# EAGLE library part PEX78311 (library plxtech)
PCI Express Endpoint Interface Auto generated by make-symbol-device-package-bsdl.ulp Rev. 16 from PEX8311_BSDL_netlist_r1.0.dat and manuell corrected Source: PEX_8311AA_Data_Book_v0.90_10Apr06.pdf
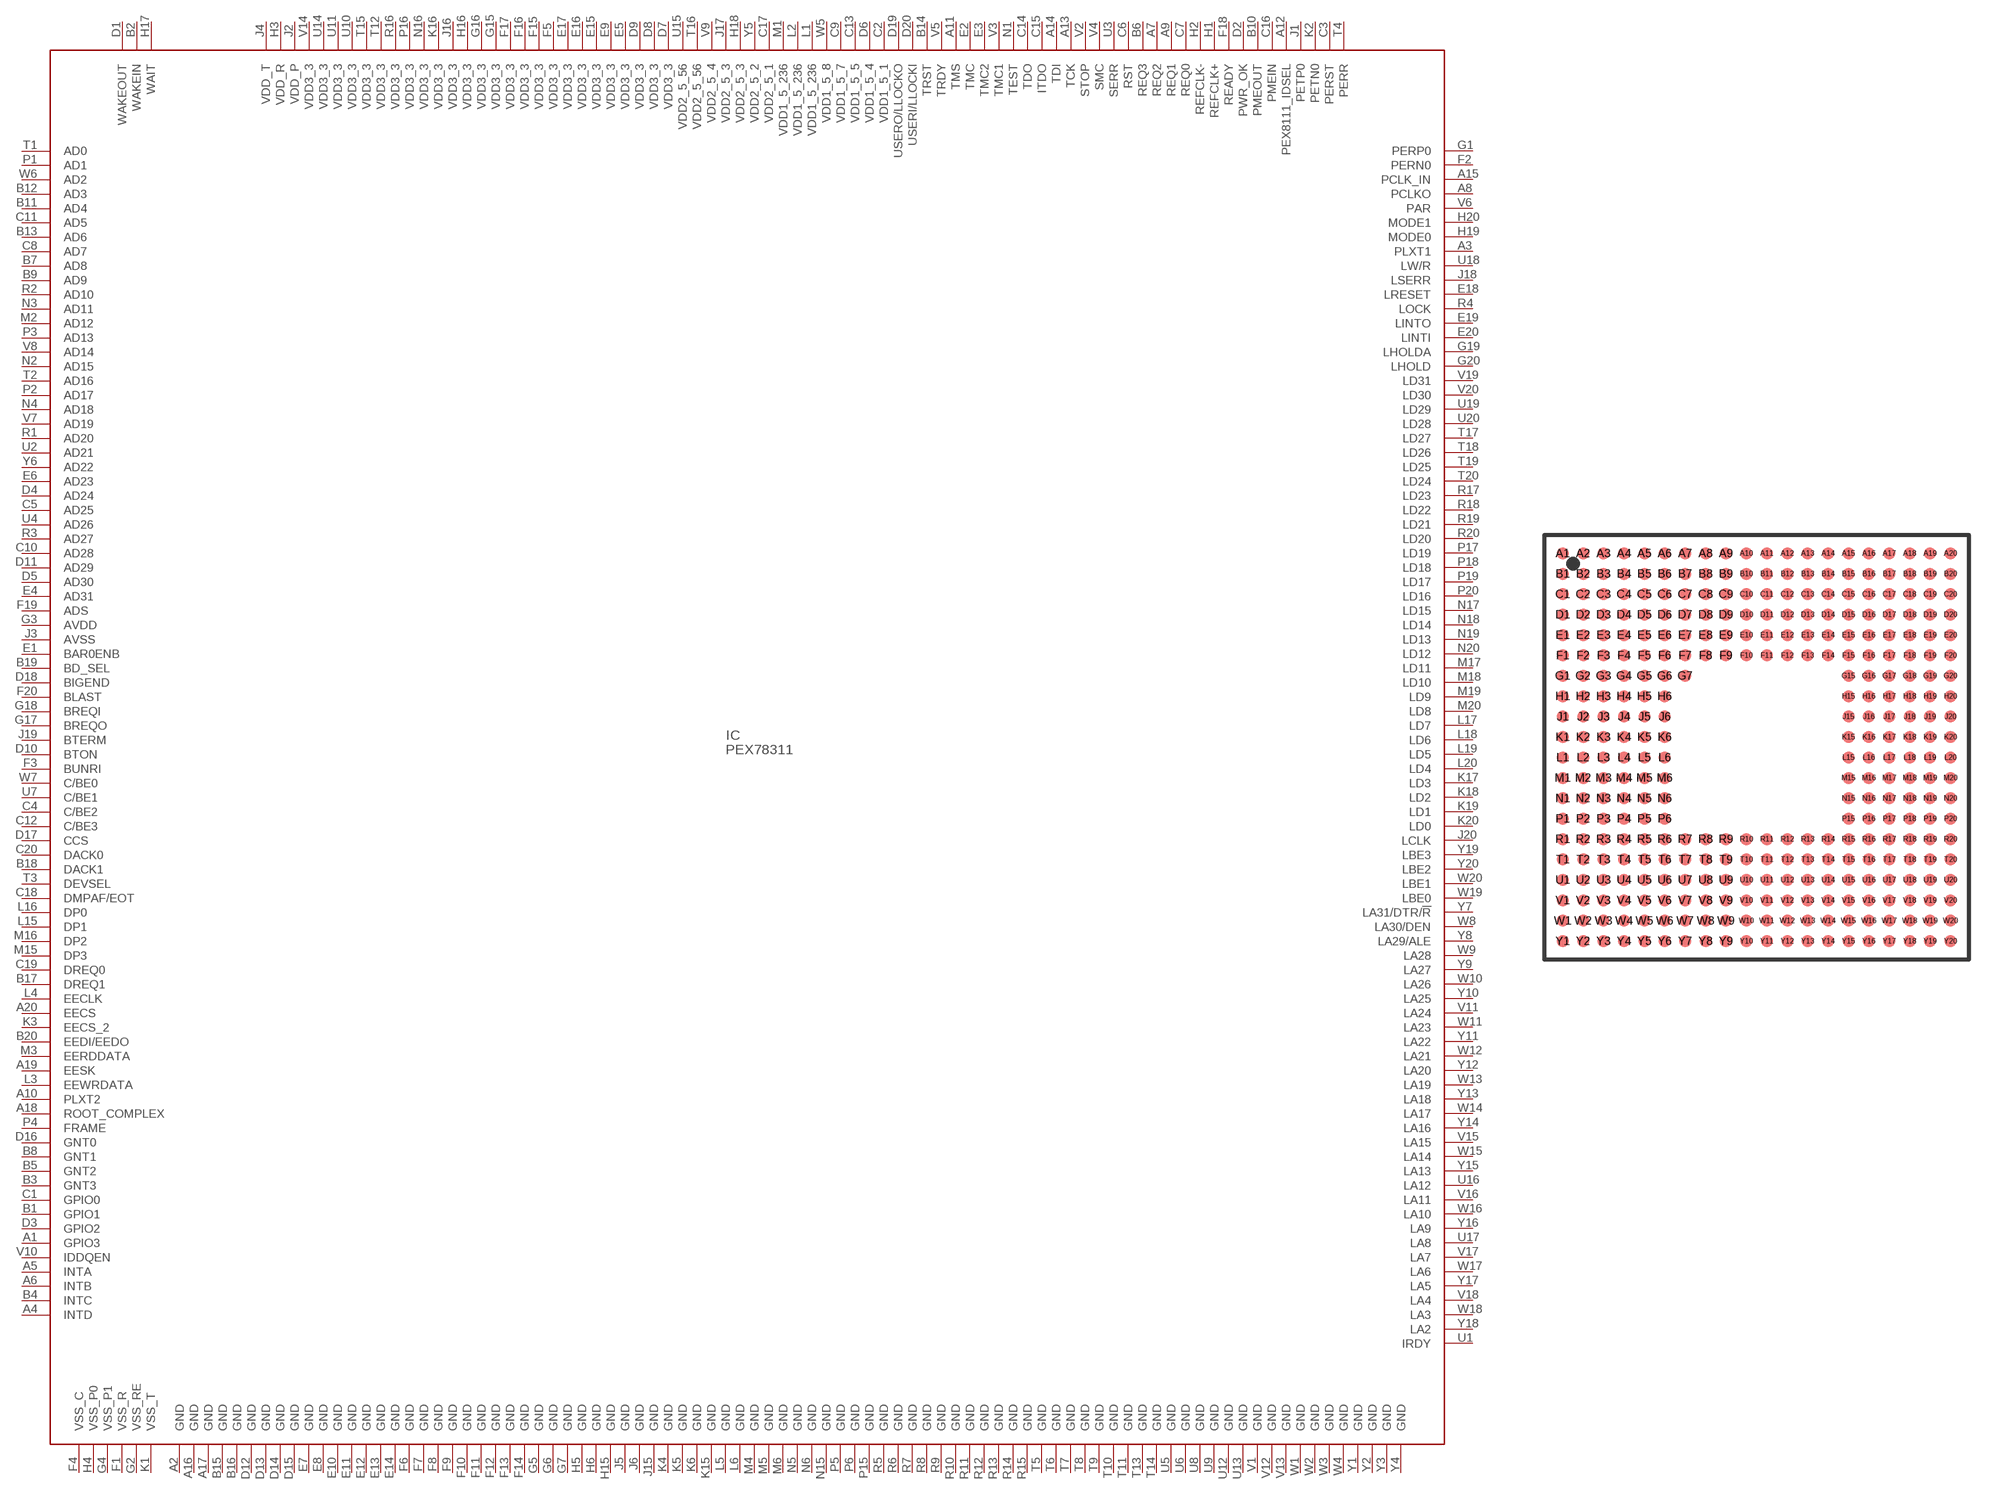
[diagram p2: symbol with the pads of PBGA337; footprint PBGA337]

Designator prefix IC

## PEX78311 (OC_FARNELL: unknown; OC_NEWARK: unknown)  [PBGA337]
A1  GPIO3
A2  GND  pwr
A3  PLXT1  in
A4  INTD
A5  INTA
A6  INTB
A7  REQ2
A8  PCLKO  out
A9  REQ1
A10  PLXT2  in
A11  TMS  in
A12  PEX8111_IDSEL
A13  TCK  in
A14  TDI  in
A15  PCLK_IN  in
A16  GND  pwr
A17  GND  pwr
A18  ROOT_COMPLEX  in
A19  EESK  out
A20  EECS  out
B1  GPIO1
B2  WAKEIN  in
B3  GNT3
B4  INTC
B5  GNT2
B6  REQ3
B7  AD8
B8  GNT1
B9  AD9
B10  PMEOUT  out
B11  AD4
B12  AD3
B13  AD6
B14  TRST  in
B15  GND  pwr
B16  GND  pwr
B17  DREQ1  in
B18  DACK1  out
B19  BD_SEL  in
B20  EEDI/EEDO
C1  GPIO0
C2  VDD1_5_1  pwr
C3  PERST
C4  C/BE2
C5  AD25
C6  RST
C7  REQ0
C8  AD7
C9  VDD1_5_7  pwr
C10  AD28
C11  AD5
C12  C/BE3
C13  VDD1_5_5  pwr
C14  TDO  out
C15  ITDO
C16  PMEIN  in
C17  VDD2_5_1  pwr
C18  DMPAF/EOT
C19  DREQ0  in
C20  DACK0  out
D1  WAKEOUT  out
D2  PWR_OK  out
D3  GPIO2
D4  AD24
D5  AD30
D6  VDD1_5_4  pwr
D7  VDD3_3  pwr
D8  VDD3_3  pwr
D9  VDD3_3  pwr
D10  BTON  in
D11  AD29
D12  GND  pwr
D13  GND  pwr
D14  GND  pwr
D15  GND  pwr
D16  GNT0
D17  CCS  in
D18  BIGEND  in
D19  USERO/LLOCKO  out
D20  USERI/LLOCKI  in
E1  BAR0ENB  in
E2  TMC  in
E3  TMC2  in
E4  AD31
E5  VDD3_3  pwr
E6  AD23
E7  GND  pwr
E8  GND  pwr
E9  VDD3_3  pwr
E10  GND  pwr
E11  GND  pwr
E12  GND  pwr
E13  GND  pwr
E14  GND  pwr
E15  VDD3_3  pwr
E16  VDD3_3  pwr
E17  VDD3_3  pwr
E18  LRESET
E19  LINTO  out
E20  LINTI  in
F1  VSS_R  pwr
F2  PERN0  in
F3  BUNRI  in
F4  VSS_C  pwr
F5  VDD3_3  pwr
F6  GND  pwr
F7  GND  pwr
F8  GND  pwr
F9  GND  pwr
F10  GND  pwr
F11  GND  pwr
F12  GND  pwr
F13  GND  pwr
F14  GND  pwr
F15  VDD3_3  pwr
F16  VDD3_3  pwr
F17  VDD3_3  pwr
F18  READY
F19  ADS
F20  BLAST
G1  PERP0  in
G2  VSS_RE  pwr
G3  AVDD  pwr
G4  VSS_P1  pwr
G5  GND  pwr
G6  GND  pwr
G7  GND  pwr
G15  VDD3_3  pwr
G16  VDD3_3  pwr
G17  BREQO  out
G18  BREQI  in
G19  LHOLDA  in
G20  LHOLD  out
H1  REFCLK+  in
H2  REFCLK-  in
H3  VDD_R  pwr
H4  VSS_P0  pwr
H5  GND  pwr
H6  GND  pwr
H15  GND  pwr
H16  VDD3_3  pwr
H17  WAIT
H18  VDD2_5_3  pwr
H19  MODE0  in
H20  MODE1  in
J1  PETP0  out
J2  VDD_P  pwr
J3  AVSS  pwr
J4  VDD_T  pwr
J5  GND  pwr
J6  GND  pwr
J15  GND  pwr
J16  VDD3_3  pwr
J17  VDD2_5_3  pwr
J18  LSERR  out
J19  BTERM
J20  LCLK  in
K1  VSS_T  pwr
K2  PETN0  out
K3  EECS_2
K4  GND  pwr
K5  GND  pwr
K6  GND  pwr
K15  GND  pwr
K16  VDD3_3  pwr
K17  LD3
K18  LD2
K19  LD1
K20  LD0
L1  VDD1_5_236  pwr
L2  VDD1_5_236  pwr
L3  EEWRDATA
L4  EECLK  out
L5  GND  pwr
L6  GND  pwr
L15  DP1
L16  DP0
L17  LD7
L18  LD6
L19  LD5
L20  LD4
M1  VDD1_5_236  pwr
M2  AD12
M3  EERDDATA  out
M4  GND  pwr
M5  GND  pwr
M6  GND  pwr
M15  DP3
M16  DP2
M17  LD11
M18  LD10
M19  LD9
M20  LD8
N1  TEST  in
N2  AD15
N3  AD11
N4  AD18
N5  GND  pwr
N6  GND  pwr
N15  GND  pwr
N16  VDD3_3  pwr
N17  LD15
N18  LD14
N19  LD13
N20  LD12
P1  AD1
P2  AD17
P3  AD13
P4  FRAME
P5  GND  pwr
P6  GND  pwr
P15  GND  pwr
P16  VDD3_3  pwr
P17  LD19
P18  LD18
P19  LD17
P20  LD16
R1  AD20
R2  AD10
R3  AD27
R4  LOCK
R5  GND  pwr
R6  GND  pwr
R7  GND  pwr
R8  GND  pwr
R9  GND  pwr
R10  GND  pwr
R11  GND  pwr
R12  GND  pwr
R13  GND  pwr
R14  GND  pwr
R15  GND  pwr
R16  VDD3_3  pwr
R17  LD23
R18  LD22
R19  LD21
R20  LD20
T1  AD0
T2  AD16
T3  DEVSEL
T4  PERR
T5  GND  pwr
T6  GND  pwr
T7  GND  pwr
T8  GND  pwr
T9  GND  pwr
T10  GND  pwr
T11  GND  pwr
T12  VDD3_3  pwr
T13  GND  pwr
T14  GND  pwr
T15  VDD3_3  pwr
T16  VDD2_5_56  pwr
T17  LD27
T18  LD26
T19  LD25
T20  LD24
U1  IRDY
U2  AD21
U3  SERR
U4  AD26
U5  GND  pwr
U6  GND  pwr
U7  C/BE1
U8  GND  pwr
U9  GND  pwr
U10  VDD3_3  pwr
U11  VDD3_3  pwr
U12  GND  pwr
U13  GND  pwr
U14  VDD3_3  pwr
U15  VDD2_5_56  pwr
U16  LA12
U17  LA8
U18  LW/R
U19  LD29
U20  LD28
V1  GND  pwr
V2  STOP
V3  TMC1  in
V4  SMC  in
V5  TRDY
V6  PAR
V7  AD19
V8  AD14
V9  VDD2_5_4  pwr
V10  IDDQEN  in
V11  LA24
V12  GND  pwr
V13  GND  pwr
V14  VDD3_3  pwr
V15  LA15
V16  LA11
V17  LA7
V18  LA4
V19  LD31
V20  LD30
W1  GND  pwr
W2  GND  pwr
W3  GND  pwr
W4  GND  pwr
W5  VDD1_5_8  pwr
W6  AD2
W7  C/BE0
W8  LA30/DEN
W9  LA28
W10  LA26
W11  LA23
W12  LA21
W13  LA19
W14  LA17
W15  LA14
W16  LA10
W17  LA6
W18  LA3
W19  LBE0
W20  LBE1
Y1  GND  pwr
Y2  GND  pwr
Y3  GND  pwr
Y4  GND  pwr
Y5  VDD2_5_2  pwr
Y6  AD22
Y7  LA31/DTR/!R
Y8  LA29/ALE
Y9  LA27
Y10  LA25
Y11  LA22
Y12  LA20
Y13  LA18
Y14  LA16
Y15  LA13
Y16  LA9
Y17  LA5
Y18  LA2
Y19  LBE3
Y20  LBE2

## Footprint PBGA337 (pad centres in mm)
PEX 8311 337-Ball PBGA Package Source: www.plxtech.com ... PEX_8311AA_Data_Book_v0.90_10Apr06.pdf
smd 0.6 x 0.6: A1 -9.5,9.5; A2 -8.5,9.5; A3 -7.5,9.5; A4 -6.5,9.5; A5 -5.5,9.5; A6 -4.5,9.5; A7 -3.5,9.5; A8 -2.5,9.5; A9 -1.5,9.5; A10 -0.5,9.5; A11 0.5,9.5; A12 1.5,9.5; A13 2.5,9.5; A14 3.5,9.5; A15 4.5,9.5; A16 5.5,9.5; A17 6.5,9.5; A18 7.5,9.5; A19 8.5,9.5; A20 9.5,9.5; B1 -9.5,8.5; B2 -8.5,8.5; B3 -7.5,8.5; B4 -6.5,8.5; B5 -5.5,8.5; B6 -4.5,8.5; B7 -3.5,8.5; B8 -2.5,8.5; B9 -1.5,8.5; B10 -0.5,8.5; B11 0.5,8.5; B12 1.5,8.5; B13 2.5,8.5; B14 3.5,8.5; B15 4.5,8.5; B16 5.5,8.5; B17 6.5,8.5; B18 7.5,8.5; B19 8.5,8.5; B20 9.5,8.5; C1 -9.5,7.5; C2 -8.5,7.5; C3 -7.5,7.5; C4 -6.5,7.5; C5 -5.5,7.5; C6 -4.5,7.5; C7 -3.5,7.5; C8 -2.5,7.5; C9 -1.5,7.5; C10 -0.5,7.5; C11 0.5,7.5; C12 1.5,7.5; C13 2.5,7.5; C14 3.5,7.5; C15 4.5,7.5; C16 5.5,7.5; C17 6.5,7.5; C18 7.5,7.5; C19 8.5,7.5; C20 9.5,7.5; D1 -9.5,6.5; D2 -8.5,6.5; D3 -7.5,6.5; D4 -6.5,6.5; D5 -5.5,6.5; D6 -4.5,6.5; D7 -3.5,6.5; D8 -2.5,6.5; D9 -1.5,6.5; D10 -0.5,6.5; D11 0.5,6.5; D12 1.5,6.5; D13 2.5,6.5; D14 3.5,6.5; D15 4.5,6.5; D16 5.5,6.5; D17 6.5,6.5; D18 7.5,6.5; D19 8.5,6.5; D20 9.5,6.5; E1 -9.5,5.5; E2 -8.5,5.5; E3 -7.5,5.5; E4 -6.5,5.5; E5 -5.5,5.5; E6 -4.5,5.5; E7 -3.5,5.5; E8 -2.5,5.5; E9 -1.5,5.5; E10 -0.5,5.5; E11 0.5,5.5; E12 1.5,5.5; E13 2.5,5.5; E14 3.5,5.5; E15 4.5,5.5; E16 5.5,5.5; E17 6.5,5.5; E18 7.5,5.5; E19 8.5,5.5; E20 9.5,5.5; F1 -9.5,4.5; F2 -8.5,4.5; F3 -7.5,4.5; F4 -6.5,4.5; F5 -5.5,4.5; F6 -4.5,4.5; F7 -3.5,4.5; F8 -2.5,4.5; F9 -1.5,4.5; F10 -0.5,4.5; F11 0.5,4.5; F12 1.5,4.5; F13 2.5,4.5; F14 3.5,4.5; F15 4.5,4.5; F16 5.5,4.5; F17 6.5,4.5; F18 7.5,4.5; F19 8.5,4.5; F20 9.5,4.5; G1 -9.5,3.5; G2 -8.5,3.5; G3 -7.5,3.5; G4 -6.5,3.5; G5 -5.5,3.5; G6 -4.5,3.5; G7 -3.5,3.5; G15 4.5,3.5; G16 5.5,3.5; G17 6.5,3.5; G18 7.5,3.5; G19 8.5,3.5; G20 9.5,3.5; H1 -9.5,2.5; H2 -8.5,2.5; H3 -7.5,2.5; H4 -6.5,2.5; H5 -5.5,2.5; H6 -4.5,2.5; H15 4.5,2.5; H16 5.5,2.5; H17 6.5,2.5; H18 7.5,2.5; H19 8.5,2.5; H20 9.5,2.5; J1 -9.5,1.5; J2 -8.5,1.5; J3 -7.5,1.5; J4 -6.5,1.5; J5 -5.5,1.5; J6 -4.5,1.5; J15 4.5,1.5; J16 5.5,1.5; J17 6.5,1.5; J18 7.5,1.5; J19 8.5,1.5; J20 9.5,1.5; K1 -9.5,0.5; K2 -8.5,0.5; K3 -7.5,0.5; K4 -6.5,0.5; K5 -5.5,0.5; K6 -4.5,0.5; K15 4.5,0.5; K16 5.5,0.5; K17 6.5,0.5; K18 7.5,0.5; K19 8.5,0.5; K20 9.5,0.5; L1 -9.5,-0.5; L2 -8.5,-0.5; L3 -7.5,-0.5; L4 -6.5,-0.5; L5 -5.5,-0.5; L6 -4.5,-0.5; L15 4.5,-0.5; L16 5.5,-0.5; L17 6.5,-0.5; L18 7.5,-0.5; L19 8.5,-0.5; L20 9.5,-0.5; M1 -9.5,-1.5; M2 -8.5,-1.5; M3 -7.5,-1.5; M4 -6.5,-1.5; M5 -5.5,-1.5; M6 -4.5,-1.5; M15 4.5,-1.5; M16 5.5,-1.5; M17 6.5,-1.5; M18 7.5,-1.5; M19 8.5,-1.5; M20 9.5,-1.5; N1 -9.5,-2.5; N2 -8.5,-2.5; N3 -7.5,-2.5; N4 -6.5,-2.5; N5 -5.5,-2.5; N6 -4.5,-2.5; N15 4.5,-2.5; N16 5.5,-2.5; N17 6.5,-2.5; N18 7.5,-2.5; N19 8.5,-2.5; N20 9.5,-2.5; P1 -9.5,-3.5; P2 -8.5,-3.5; P3 -7.5,-3.5; P4 -6.5,-3.5; P5 -5.5,-3.5; P6 -4.5,-3.5; P15 4.5,-3.5; P16 5.5,-3.5; P17 6.5,-3.5; P18 7.5,-3.5; P19 8.5,-3.5; P20 9.5,-3.5; R1 -9.5,-4.5; R2 -8.5,-4.5; R3 -7.5,-4.5; R4 -6.5,-4.5; R5 -5.5,-4.5; R6 -4.5,-4.5; R7 -3.5,-4.5; R8 -2.5,-4.5; R9 -1.5,-4.5; R10 -0.5,-4.5; R11 0.5,-4.5; R12 1.5,-4.5; R13 2.5,-4.5; R14 3.5,-4.5; R15 4.5,-4.5; R16 5.5,-4.5; R17 6.5,-4.5; R18 7.5,-4.5; R19 8.5,-4.5; R20 9.5,-4.5; T1 -9.5,-5.5; T2 -8.5,-5.5; T3 -7.5,-5.5; T4 -6.5,-5.5; T5 -5.5,-5.5; T6 -4.5,-5.5; T7 -3.5,-5.5; T8 -2.5,-5.5; T9 -1.5,-5.5; T10 -0.5,-5.5; T11 0.5,-5.5; T12 1.5,-5.5; T13 2.5,-5.5; T14 3.5,-5.5; T15 4.5,-5.5; T16 5.5,-5.5; T17 6.5,-5.5; T18 7.5,-5.5; T19 8.5,-5.5; T20 9.5,-5.5; U1 -9.5,-6.5; U2 -8.5,-6.5; U3 -7.5,-6.5; U4 -6.5,-6.5; U5 -5.5,-6.5; U6 -4.5,-6.5; U7 -3.5,-6.5; U8 -2.5,-6.5; U9 -1.5,-6.5; U10 -0.5,-6.5; U11 0.5,-6.5; U12 1.5,-6.5; U13 2.5,-6.5; U14 3.5,-6.5; U15 4.5,-6.5; U16 5.5,-6.5; U17 6.5,-6.5; U18 7.5,-6.5; U19 8.5,-6.5; U20 9.5,-6.5; V1 -9.5,-7.5; V2 -8.5,-7.5; V3 -7.5,-7.5; V4 -6.5,-7.5; V5 -5.5,-7.5; V6 -4.5,-7.5; V7 -3.5,-7.5; V8 -2.5,-7.5; V9 -1.5,-7.5; V10 -0.5,-7.5; V11 0.5,-7.5; V12 1.5,-7.5; V13 2.5,-7.5; V14 3.5,-7.5; V15 4.5,-7.5; V16 5.5,-7.5; V17 6.5,-7.5; V18 7.5,-7.5; V19 8.5,-7.5; V20 9.5,-7.5; W1 -9.5,-8.5; W2 -8.5,-8.5; W3 -7.5,-8.5; W4 -6.5,-8.5; W5 -5.5,-8.5; W6 -4.5,-8.5; W7 -3.5,-8.5; W8 -2.5,-8.5; W9 -1.5,-8.5; W10 -0.5,-8.5; W11 0.5,-8.5; W12 1.5,-8.5; W13 2.5,-8.5; W14 3.5,-8.5; W15 4.5,-8.5; W16 5.5,-8.5; W17 6.5,-8.5; W18 7.5,-8.5; W19 8.5,-8.5; W20 9.5,-8.5; Y1 -9.5,-9.5; Y2 -8.5,-9.5; Y3 -7.5,-9.5; Y4 -6.5,-9.5; Y5 -5.5,-9.5; Y6 -4.5,-9.5; Y7 -3.5,-9.5; Y8 -2.5,-9.5; Y9 -1.5,-9.5; Y10 -0.5,-9.5; Y11 0.5,-9.5; Y12 1.5,-9.5; Y13 2.5,-9.5; Y14 3.5,-9.5; Y15 4.5,-9.5; Y16 5.5,-9.5; Y17 6.5,-9.5; Y18 7.5,-9.5; Y19 8.5,-9.5; Y20 9.5,-9.5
